ORGANIZATION_BLOCK "Ciclo"
TITLE = "Main Program Sweep (Cycle)"
VERSION : 0.1


VAR_TEMP
  OB1_EV_CLASS : BYTE ;	//Bits 0-3 = 1 (Coming event), Bits 4-7 = 1 (Event class 1)
  OB1_SCAN_1 : BYTE ;	//1 (Cold restart scan 1 of OB 1), 3 (Scan 2-n of OB 1)
  OB1_PRIORITY : BYTE ;	//1 (Priority of 1 is lowest)
  OB1_OB_NUMBR : BYTE ;	//1 (Organization block 1, OB1)
  OB1_RESERVED_1 : BYTE ;	//Reserved for system
  OB1_RESERVED_2 : BYTE ;	//Reserved for system
  OB1_PREV_CYCLE : INT ;	//Cycle time of previous OB1 scan (milliseconds)
  OB1_MIN_CYCLE : INT ;	//Minimum cycle time of OB1 (milliseconds)
  OB1_MAX_CYCLE : INT ;	//Maximum cycle time of OB1 (milliseconds)
  OB1_DATE_TIME : DATE_AND_TIME ;	//Date and time OB1 started
END_VAR
BEGIN
NETWORK
TITLE =


      UC    "Emergenze";
      UC    "GestioneFronti";
      UC    "GestioneTimer";
      UC    "ModiDiFunzionamento";
      UC    "CicloAutomatico";
      UC    "CicloManuali";
      UC    "CicloAzzeramento";
      UC    "CicloEspulsore";
      UC    "Uscite";
      UC    "CicloResetAllarmi";
      UC    "CicloEspulsore";
      UC    "ScambioSegnaliProfi";

NETWORK
TITLE =

      CALL "DIVE" ;

NETWORK
TITLE =



END_ORGANIZATION_BLOCK

